(* SV publisher APDU *)
{attribute 'analysis' := '-33'}
{attribute 'no_assign'}
{attribute 'no_explicit_call' := 'Direct call not allowed for type FB_SVTXAPDU_IED_MUnn_LLN0_MSVCB01'}
FUNCTION_BLOCK FB_SVTXAPDU_IED_MUnn_LLN0_MSVCB01 EXTENDS FB_GseSvApduClass
VAR_INPUT
	TxData: ST_SVAPDU_IED_MUnn_LLN0_MSVCB01; (* SV data to be published in TwinCAT PLC host format (little endian) *)
END_VAR
VAR
	Asdu1: FB_SVTXASDU_IED_MUnn_LLN0_MSVCB01 := (index:=0, ipApdu:=THIS^.AddAsduToContainer(ipAsdu:=Asdu1)); (* Adds ASDU to APDU *)
END_VAR

{attribute 'analysis' := '-33'}
(* Converts SV publisher data to be sent from host (little-endian) to network (big-endian) byte order *)
METHOD FINAL OnSvPublisherHostToNet
VAR_INPUT
	ipAdapter: I_GseAdapterClass; (* Network adapter interface pointer *)
	ipApdu: I_GseSvApduClass; (* APDU object interface pointer *)
END_VAR
VAR
END_VAR
Asdu1.nSmpCnt:= TxData.Asdu1.nSmpCnt; (* Set sample counter *)
Asdu1.eSmpSynch:= TxData.Asdu1.eSmpSynch; (* Set synchronization type: 0..2 *)
Asdu1.tRefrTm:= TxData.Asdu1.tRefrTm; (* Set refresh time stamp (optional) *)

(* Convert SV data to be sent from host byte order to network byte order *)
HostToNetInt32(in:=TxData.Asdu1.IED_MUnn_InnATCTR1_AmpSv_instMag_i, out:=Asdu1.Values.IED_MUnn_InnATCTR1_AmpSv_instMag_i);
HostToNetQuality(in:=TxData.Asdu1.IED_MUnn_InnATCTR1_AmpSv_q, out:=Asdu1.Values.IED_MUnn_InnATCTR1_AmpSv_q);
HostToNetInt32(in:=TxData.Asdu1.IED_MUnn_InnBTCTR2_AmpSv_instMag_i, out:=Asdu1.Values.IED_MUnn_InnBTCTR2_AmpSv_instMag_i);
HostToNetQuality(in:=TxData.Asdu1.IED_MUnn_InnBTCTR2_AmpSv_q, out:=Asdu1.Values.IED_MUnn_InnBTCTR2_AmpSv_q);
HostToNetInt32(in:=TxData.Asdu1.IED_MUnn_InnCTCTR3_AmpSv_instMag_i, out:=Asdu1.Values.IED_MUnn_InnCTCTR3_AmpSv_instMag_i);
HostToNetQuality(in:=TxData.Asdu1.IED_MUnn_InnCTCTR3_AmpSv_q, out:=Asdu1.Values.IED_MUnn_InnCTCTR3_AmpSv_q);
HostToNetInt32(in:=TxData.Asdu1.IED_MUnn_InnNTCTR4_AmpSv_instMag_i, out:=Asdu1.Values.IED_MUnn_InnNTCTR4_AmpSv_instMag_i);
HostToNetQuality(in:=TxData.Asdu1.IED_MUnn_InnNTCTR4_AmpSv_q, out:=Asdu1.Values.IED_MUnn_InnNTCTR4_AmpSv_q);
HostToNetInt32(in:=TxData.Asdu1.IED_MUnn_UnnATVTR1_VolSv_instMag_i, out:=Asdu1.Values.IED_MUnn_UnnATVTR1_VolSv_instMag_i);
HostToNetQuality(in:=TxData.Asdu1.IED_MUnn_UnnATVTR1_VolSv_q, out:=Asdu1.Values.IED_MUnn_UnnATVTR1_VolSv_q);
HostToNetInt32(in:=TxData.Asdu1.IED_MUnn_UnnBTVTR2_VolSv_instMag_i, out:=Asdu1.Values.IED_MUnn_UnnBTVTR2_VolSv_instMag_i);
HostToNetQuality(in:=TxData.Asdu1.IED_MUnn_UnnBTVTR2_VolSv_q, out:=Asdu1.Values.IED_MUnn_UnnBTVTR2_VolSv_q);
HostToNetInt32(in:=TxData.Asdu1.IED_MUnn_UnnCTVTR3_VolSv_instMag_i, out:=Asdu1.Values.IED_MUnn_UnnCTVTR3_VolSv_instMag_i);
HostToNetQuality(in:=TxData.Asdu1.IED_MUnn_UnnCTVTR3_VolSv_q, out:=Asdu1.Values.IED_MUnn_UnnCTVTR3_VolSv_q);
HostToNetInt32(in:=TxData.Asdu1.IED_MUnn_UnnNTVTR4_VolSv_instMag_i, out:=Asdu1.Values.IED_MUnn_UnnNTVTR4_VolSv_instMag_i);
HostToNetQuality(in:=TxData.Asdu1.IED_MUnn_UnnNTVTR4_VolSv_q, out:=Asdu1.Values.IED_MUnn_UnnNTVTR4_VolSv_q);
END_METHOD

END_FUNCTION_BLOCK
